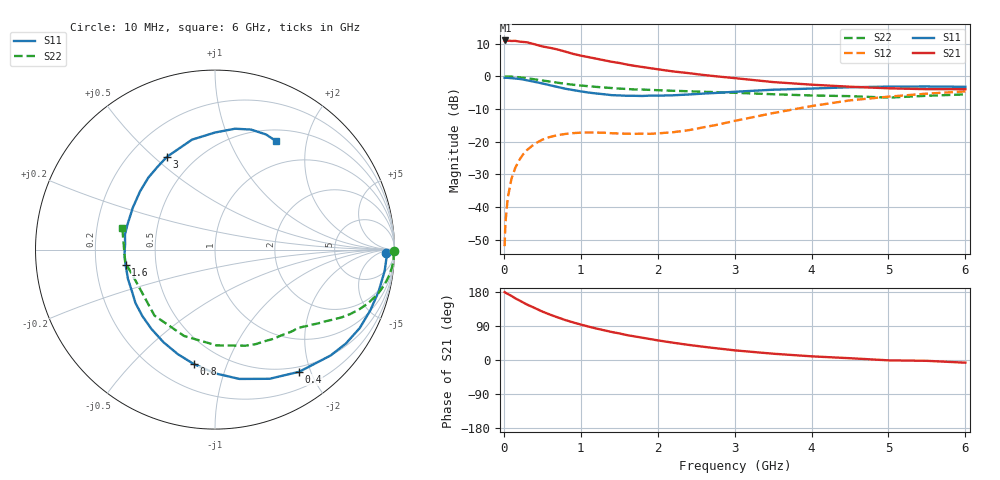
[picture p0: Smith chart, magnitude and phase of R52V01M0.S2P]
! SIEMENS Small Signal Semiconductors
! BFR183
! Si NPN RF Bipolar Junction Transistor in SOT23
! VCE = 2 V  IC = 1 mA
! Common Emitter S-Parameters:  May  1996
# GHz  S  MA  R  50
!  f  S11  S21  S12  S22
! GHz  MAG  ANG  MAG  ANG  MAG  ANG  MAG  ANG
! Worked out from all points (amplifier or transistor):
!   36 points, 10 MHz to 6 GHz, reference 50 ohm
!   highest |S21| = 11.0 dB at 20 MHz (marker M1)
!   |S21| within 3 dB of that: start of sweep to 734.4 MHz
!   unconditionally stable (mu >= 1): 1.637 GHz to 2.953 GHz
!   at 250 MHz: K = 0.16, MSG = 17.2 dB, |S12| = -23.9 dB
!   at 1.4 GHz: K = 0.86, MSG = 11.0 dB, |S12| = -17.4 dB
!   at 6 GHz: K = 0.96, MSG = 0.3 dB, |S12| = -4.6 dB
!   S11 on the Smith chart (normalised r, x): 10 MHz: 35, -17; 400 MHz: 0.43, -1.83; 800 MHz: 0.35, -0.77; 1.6 GHz: 0.33, -0.08; 3 GHz: 0.35, +0.55; 6 GHz: 0.65, +1.51
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0.01  0.9547 -1.3  3.487 179.3  0.0025 86.8  0.9989 -0.6
0.02  0.9562 -3.0  3.563 177.6  0.0055 88.7  0.9928 -1.1
0.05  0.9527 -7.2  3.543 174.4  0.0136 84.2  0.9967 -2.8
0.1  0.9408 -14.5  3.501 169.1  0.0272 81.3  0.992 -5.3
0.15  0.9291 -21.4  3.513 162.6  0.0401 76.7  0.9829 -8.1
0.3  0.8734 -42.5  3.338 146.4  0.0744 65.1  0.9401 -15.3
0.4  0.8267 -55.4  3.115 137.4  0.0925 57.9  0.9042 -19.3
0.5  0.7814 -67.1  2.885 127.9  0.1074 51.9  0.8689 -22.6
0.6  0.7334 -79.3  2.749 119.8  0.1182 46.8  0.8333 -25.6
0.7  0.6893 -90.0  2.588 112.4  0.1259 42.4  0.801 -28.1
0.8  0.648 -100.6  2.402 105.4  0.1314 38.7  0.7709 -30.2
0.9  0.6182 -109.6  2.22 99.2  0.1353 35.8  0.7463 -32.0
1.1  0.5662 -128.8  1.978 88.2  0.1382 31.5  0.7083 -35.4
1.3  0.5339 -146.1  1.774 78.6  0.1373 29.5  0.6773 -38.2
1.6  0.5054 -170.1  1.522 65.7  0.1326 30.7  0.6422 -42.6
2.2  0.5141 153.0  1.194 45.6  0.1397 43.2  0.6029 -52.8
3  0.5823 117.3  0.943 25.5  0.2085 55.5  0.5618 -72.4
3.5  0.6259 101.8  0.82 16.6  0.2743 54.1  0.5337 -89.1
4.5  0.6827 80.6  0.696 4.7  0.4301 41.0  0.4989 -132.5
5  0.6983 73.3  0.658 -0.9  0.4899 30.7  0.4737 -156.9
5.5  0.7017 66.1  0.638 -2.2  0.5451 23.9  0.5053 -172.0
6  0.6938 60.7  0.638 -7.1  0.5898 13.9  0.5309 166.7
